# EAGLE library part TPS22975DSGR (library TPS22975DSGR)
5.7V, 6A, 16m Load Switch with Adjustable Rise Time & Optional QOD for Cost-Conscious Applications Source: Datasheet
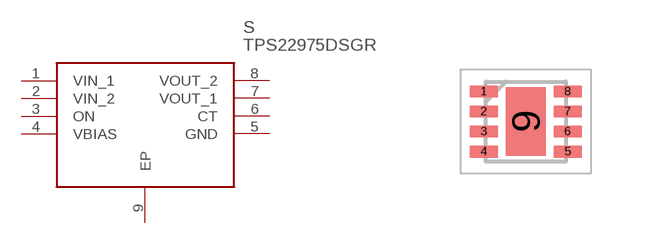
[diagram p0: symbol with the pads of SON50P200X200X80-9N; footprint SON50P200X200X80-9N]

Designator prefix S

## TPS22975DSGR (Description: 5.7V, 6A, 16m Load Switch with Adjustable Rise Time & Optional QOD for Cost-Conscious Applications; Height: 0.8mm; Manufacturer_Name: Texas Instruments; Manufacturer_Part_Number: TPS22975DSGR; Mouser_Part_Number: 595-TPS22975DSGR; Mouser_Price-Stock: https://www.mouser.co.uk/ProductDetail/Texas-Instruments/TPS22975DSGR?qs=zEmsApcVOkXVZ0HZtWdfyQ%3D%3D)  [SON50P200X200X80-9N]
1  VIN_1
2  VIN_2
3  ON
4  VBIAS
5  GND
6  CT
7  VOUT_1
8  VOUT_2
9  EP

## Footprint SON50P200X200X80-9N (pad centres in mm)
DSG0008A 1
smd 0.7 x 0.3: 1 -1.05,0.75; 2 -1.05,0.25; 3 -1.05,-0.25; 4 -1.05,-0.75; 5 1.05,-0.75; 6 1.05,-0.25; 7 1.05,0.25; 8 1.05,0.75
smd 1 x 1.7: 9 0,0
